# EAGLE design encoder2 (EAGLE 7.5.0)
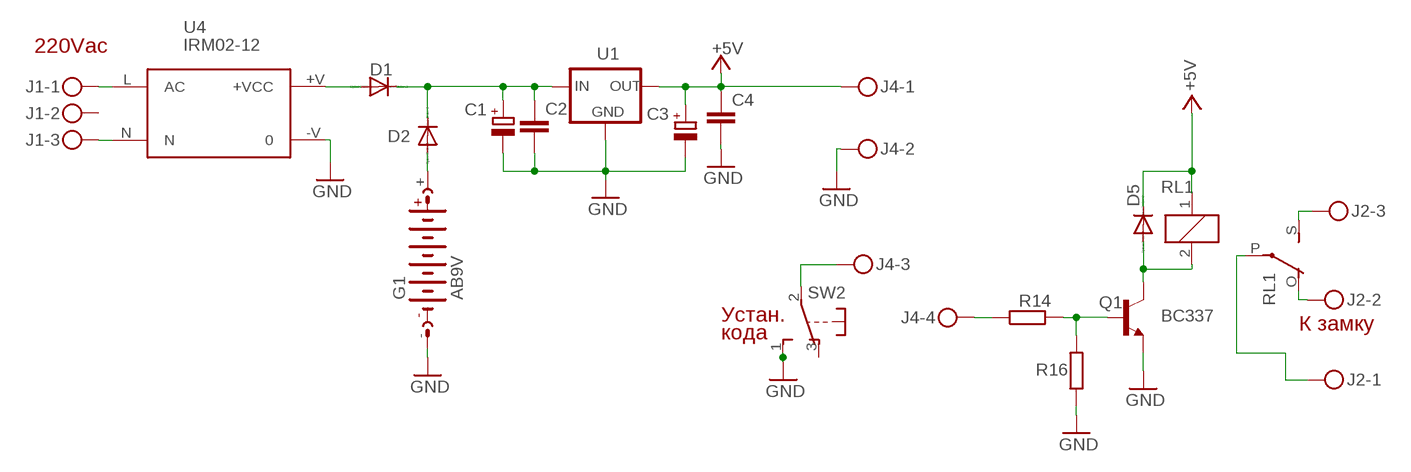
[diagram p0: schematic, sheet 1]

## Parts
C1  CPOL-EUE5-8.5  [E5-8,5]
C2  C-EUC1206  [C1206]
C3  CPOL-EUE5-8.5  [E5-8,5]
C4  C-EUC1206  [C1206]
D1  1N4004  [DO41-10]
D2  1N4004  [DO41-10]
D5  1N4004  [DO41-10]
G1  AB9V  [AB9V]
J1  MKDSN1,5/3-5,08  [MKDSN1,5/3-5,08]
J2  MKDSN1,5/3-5,08  [MKDSN1,5/3-5,08]
J4  MKDSN1,5/4-5,08  [MKDSN1,5/4-5,08]
Q1  BC337  [TO92]
R14  R-EU_0204/7  [0204/7]
R16  R-EU_0204/7  [0204/7]
RL1  G5LE  [G5LE]
SW2  9077-1  [9077-1]
U1  78XXL  [78XXL]
U4  IRM02-12  IRM02  [IRM02]

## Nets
+5V: C3.+ C4.1 D5.C J4.1 RL1.1 U1.OUT
GND: C1.- C2.2 C3.- C4.2 G1.- J4.2 Q1.1(E) R16.1 SW2.1(S) U1.GND U4.-V
N$1: J2.2 RL1.O(2:O)
N$2: J2.3 RL1.S(2:S)
N$3: J4.4 R14.1
N$4: J2.1 RL1.P(2:P)
N$5: J4.3 SW2.2(P)
N$6: Q1.2(B) R14.2 R16.2
N$8: C1.+ C2.1 D1.C D2.C U1.IN
N$9: J1.1 U4.L(AC)
N$10: J1.3 U4.N
N$11: D1.A U4.+V(+VCC)
N$12: D2.A G1.+
Q1: D5.A Q1.3(C) RL1.2
Unconnected: J1.2 SW2.3(O)

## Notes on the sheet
- 220Vac
- Устан.
- К замку
- кода

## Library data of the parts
C1 C3 = rcl:CPOL-EU: POLARIZED CAPACITOR, European symbol
C2 C4 = rcl:C-EU: CAPACITOR, European symbol
D1 D2 D5 = diode:1N4004: DIODE
G1 = battery:AB9V: 9-V BATTERY CLIP
J1 J2 = con-phoenix-508:MKDSN1,5/3-5,08: MKDSN 1,5/ 3-5,08 Printklemme Nennstrom: 13,5 A Nennspannung: 250 V Rastermaß: 5,08 mm Polzahl: 3 Anschlussart: Schraubanschluss Montage: Löten Anschlussrichtung Leiter/Platine: 0 ° Artikelnummer: 1729131 Source: http://eshop.phoenixcontact.com .. 1729131.pdf
J4 = con-phoenix-508:MKDSN1,5/4-5,08: MKDSN 1,5/ 4-5,08 Printklemme Nennstrom: 13,5 A Nennspannung: 250 V Rastermaß: 5,08 mm Polzahl: 4 Anschlussart: Schraubanschluss Montage: Löten Anschlussrichtung Leiter/Platine: 0 ° Artikelnummer: 1729144 Source: http://eshop.phoenixcontact.com .. 1729144.pdf
Q1 = transistor:BC337: NPN TRANSISTOR
R14 R16 = rcl:R-EU_: RESISTOR, European symbol
RL1 = relay:G5LE: RELAY 1 x switch, 10 A/120 V AC, 8 A/30 V DC, Omron; OC_FARNELL: unknown; OC_NEWARK: unknown
SW2 = switch-misc:9077-1: MARQUARDT SWITCH 9077.0100 Distributor: Buerklin
U1 = v-reg:78XXL: VOLTAGE REGULATOR
U4 = acdc:IRM02: 2W Single Output ACDC converter

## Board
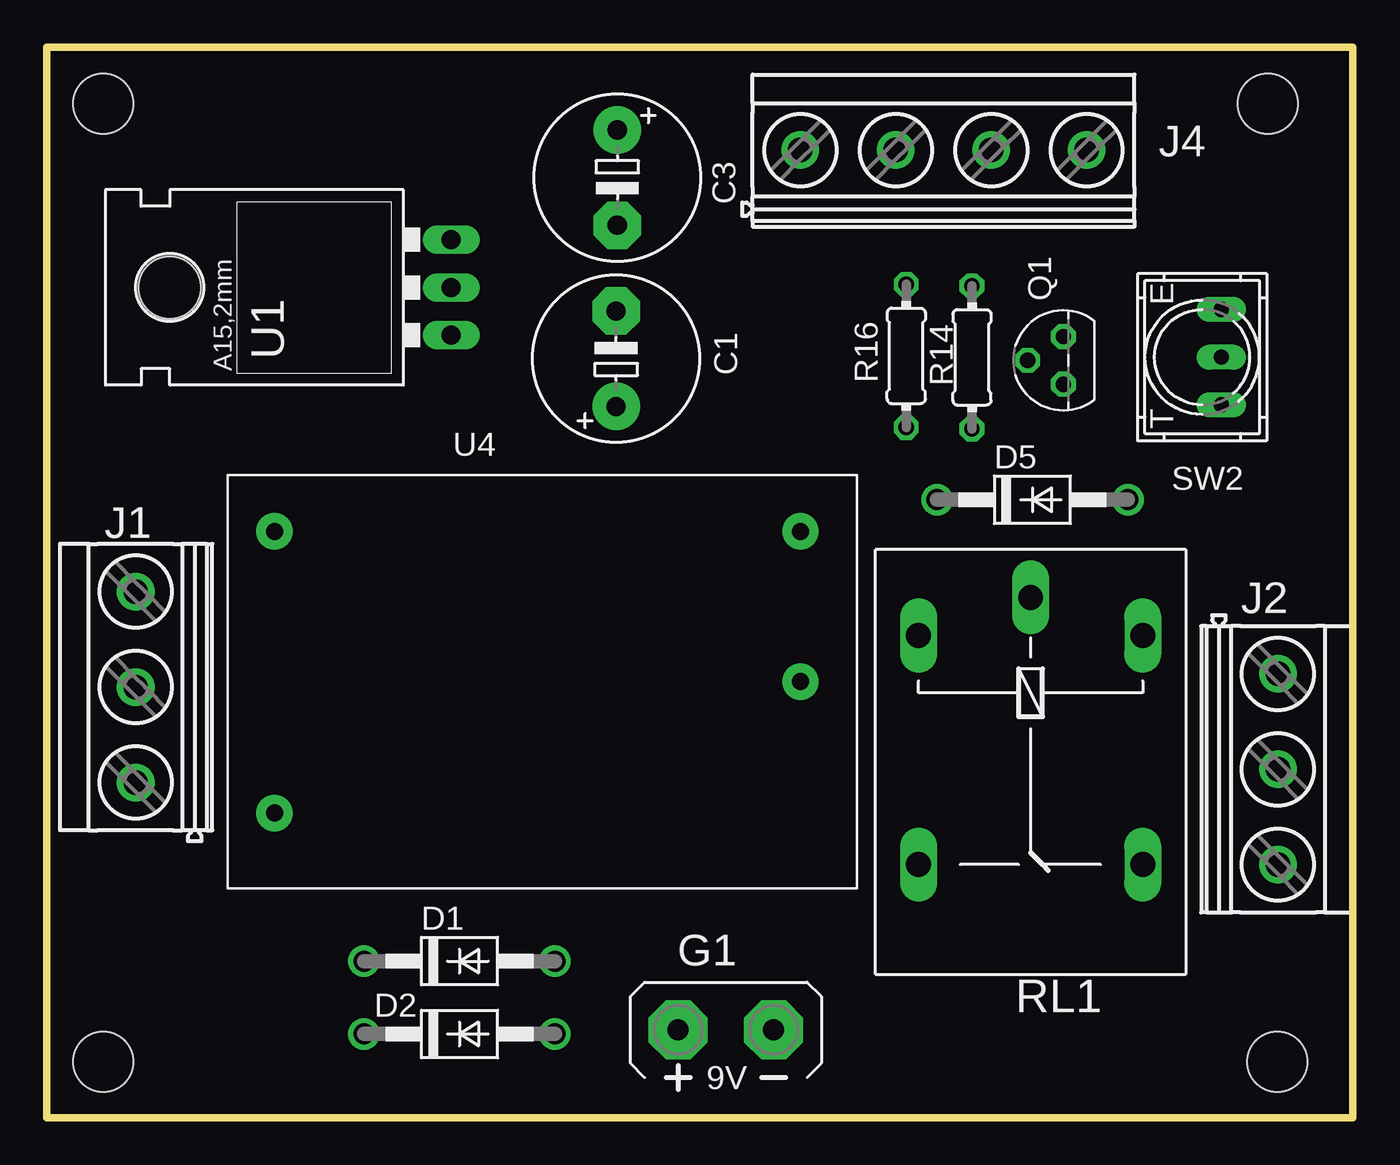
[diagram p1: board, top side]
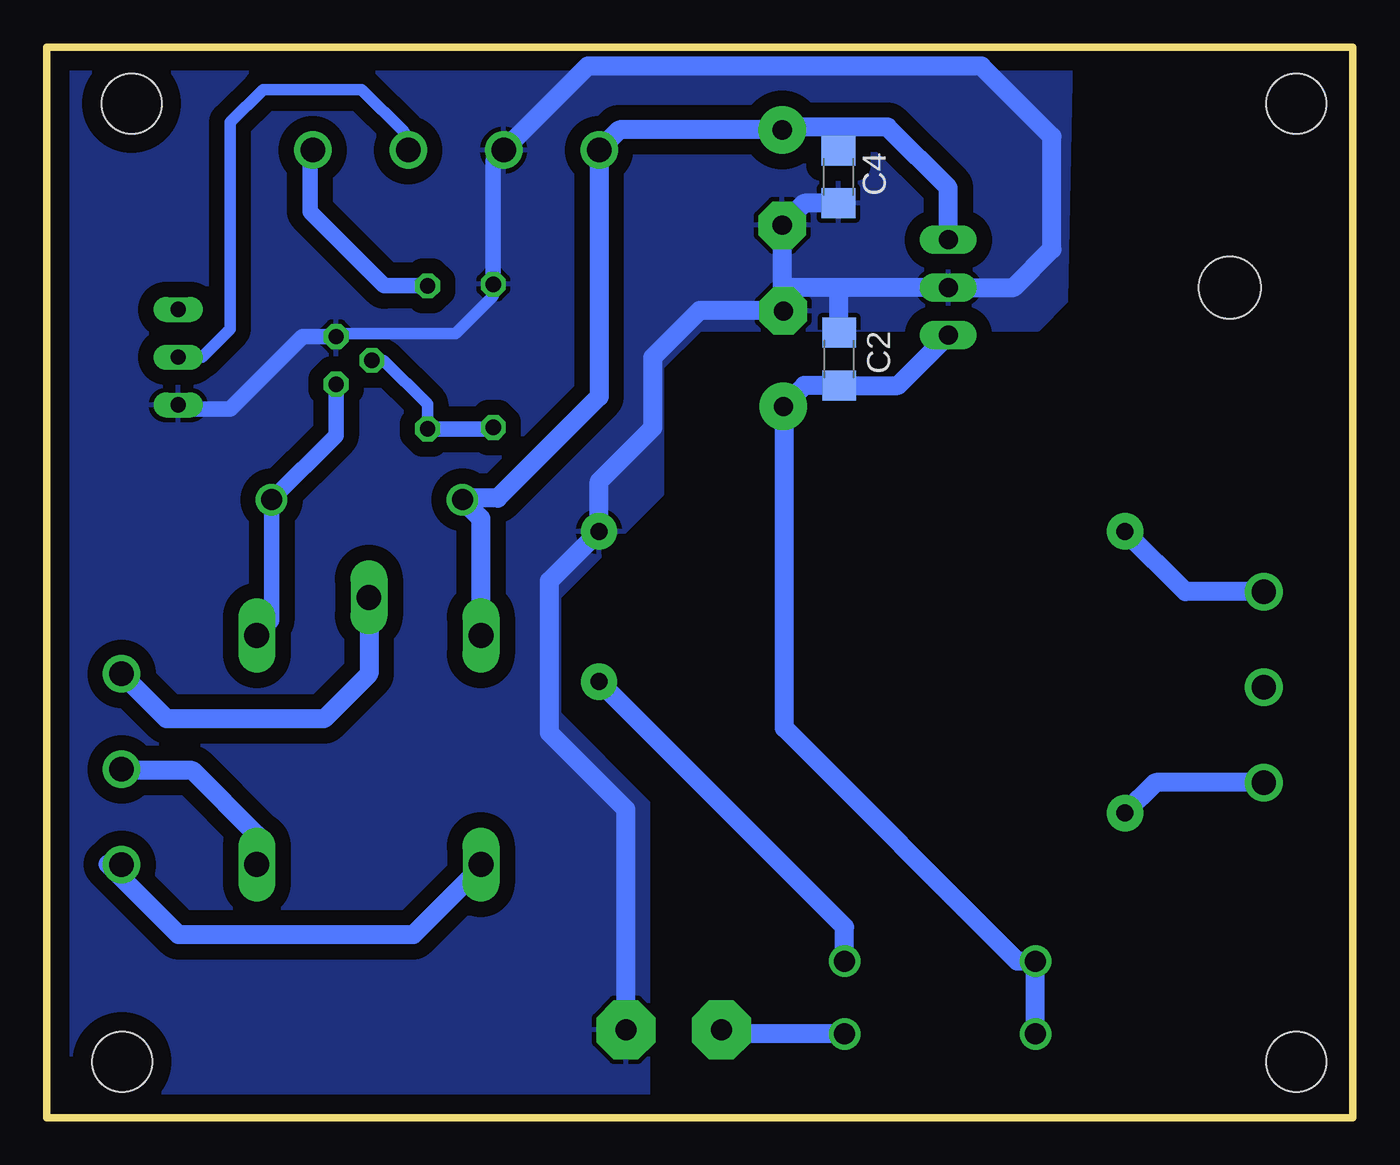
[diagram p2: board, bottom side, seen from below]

Size 69.5 x 57 mm. Coordinates in mm from the lower left corner, seen from the top.
Outline: 0,0 0,57 69.5,57 69.5,0 0,0
Copper layers (1*16): Top 0.035mm / dielectric 1.5mm / Bottom 0.035mm
Design rules "default": minimum track width 10mil, minimum drill 24mil, track to track 8mil, track to pad 8mil, pad to pad 8mil, via to via 8mil, smd to smd 8mil, copper to edge 40mil, drill to drill 8mil, minimum pad ring 10mil, minimum via ring 8mil, stop-mask expansion 4mil, vias tented up to drill 0mil, thermal gap 10mil
Holes 3.2 mm at 3,3 3,54 65,54 65.5,3

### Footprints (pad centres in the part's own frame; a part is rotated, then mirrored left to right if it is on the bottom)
E5-8,5 = drill 1.016 pad 2.54: + -2.54,0 | drill 1.016 pad 2.54 octagon: - 2.54,0
C1206 = smd 1.6 x 1.8: 1 -1.4,0; 2 1.4,0
DO41-10 = drill 1.118: A 5.08,0; C -5.08,0
AB9V = drill 1.118 pad 3.15 octagon: + 0,2.54; - 0,-2.54
MKDSN1,5/3-5,08 = drill 1.3 pad 2: 1 -7.641,0.025; 2 -2.561,0.025; 3 2.519,0.025
MKDSN1,5/4-5,08 = drill 1.3 pad 2: 1 -7.641,0.025; 2 -2.561,0.025; 3 2.519,0.025; 4 7.599,0.025
TO92 = drill 0.813 octagon: 1 1.27,0; 2 0,1.905; 3 -1.27,0
0204/7 = drill 0.813 octagon: 1 -3.81,0; 2 3.81,0
G5LE = drill 1.321 long: 1 -7.493,-5.969; 2 -7.493,5.969; O 4.699,5.969; P -9.525,0; S 4.699,-5.969
9077-1 = drill 0.813 long: 1 -2.54,-1.016; 2 0,-1.016; 3 2.54,-1.016
78XXL = drill 1.016 long: GND 0,-3.81; IN -2.54,-3.81; OUT 2.54,-3.81 | hole 3.302: 0,11.176
IRM02 = drill 0.9 pad 1.93: +V 30.5,-11; -V 30.5,-3; L 2.5,-18; N 2.5,-3

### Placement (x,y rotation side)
C1  30.3,40.42 90 top
C2  27.33,40.4 90 bottom
C3  30.36,50.06 270 top
C4  27.37,50.1 270 bottom
D1  21.96,8.35 0 top
D2  21.96,4.47 0 top
D5  52.46,32.91 0 top
G1  36.14,4.69 90 top
J1  4.75,25.5 90 top
J2  65.5,16 270 top
J4  47.75,51.5 0 top
Q1  54.11,40.33 90 top
R14  49.24,40.49 270 top
R16  45.74,40.57 270 top
RL1  52.36,18.19 270 top
SW2  61.5,40.5 90 top
U1  17.71,44.21 90 top
U4  9.61,34.23 0 top

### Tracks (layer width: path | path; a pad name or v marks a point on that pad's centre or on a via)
+5V
  Bottom 1.016: U1.OUT 21.52,49.52 24.75,52.75 27.5,52.75 | 27.5,52.75 30.21,52.75 C3.+ 39.03,52.6 J4.1 40.11,38.39 45.5,33 47.29,33 D5.C 46.39,31.92 RL1.1 | C4.1 27.37,52.62 27.5,52.75
GND
  Bottom 0.61: R16.1 45.74,43.76 47.75,41.75 53.96,41.75 Q1.1
  Bottom 0.813: Q1.1 55.9,41.6 59.75,37.75 62.31,37.75 SW2.1 | R16.1 45.74,50.97 J4.2
  Bottom 1.016: J4.2 40.71,56 19.75,56 16,52.25 16,46.25 18.04,44.21 U1.GND 27.5,44.21 | 30.36,44.25 C3.- 29.18,48.7 C4.2 | 30.36,44.25 30.36,43.02 C1.- 30.34,43 34.75,43 37.25,40.5 37.25,36.75 40.11,33.89 U4.-V 42.75,28.59 42.75,20.5 38.68,16.43 G1.- | 27.5,44.21 30.32,44.21 30.36,44.25 | C2.2 27.33,44.04 27.5,44.21
  pour Bottom (isolate 0.813): 15,56.5 69,56.5 69,0.5 37.5,0.5 37.5,16.75 42.25,21.5 42.25,27.75 36.75,33.25 36.75,40 34.75,42 16.75,42 15.25,43.5
N$1
  Bottom 1.016: RL1.O 58.33,15.08 61.75,18.5 65.46,18.5 J2.2
N$2
  Bottom 1.016: RL1.S 46.39,13.36 50,9.75 62.5,9.75 66.25,13.5 65.54,13.5 J2.3
N$3
  Bottom 0.813: R14.1 51.55,44.3 55.5,48.25 55.5,51.37 J4.4
N$4
  Bottom 1.016: RL1.P 52.36,23.64 54.75,21.25 63.13,21.25 J2.1
N$5
  Bottom 0.61: SW2.2 61.25,40.5 59.75,42 59.75,53 58,54.75 52.75,54.75 50.5,52.5 50.5,51.76 J4.3
N$6
  Bottom 0.61: Q1.2 51.58,40.33 49.25,38 R14.2
  Bottom 0.813: R14.2 45.82,36.68 R16.2
N$8
  Bottom 1.016: U1.IN 24.19,39 C2.1 29.18,39 C1.+ 30.25,37.83 30.25,20.75 17.85,8.35 D1.C D2.C
N$9
  Bottom 1.016: J1.1 10.48,17.86 U4.L
N$10
  Bottom 1.016: J1.3 8.9,28.02 U4.N
N$11
  Bottom 1.016: D1.A 27.04,10.16 U4.+V
N$12
  Bottom 1.016: D2.A 32.78,4.47 33,4.25 33.16,4.25 G1.+
Q1
  Bottom 0.813: Q1.3 54.11,36.34 D5.A 57.54,26.47 RL1.2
